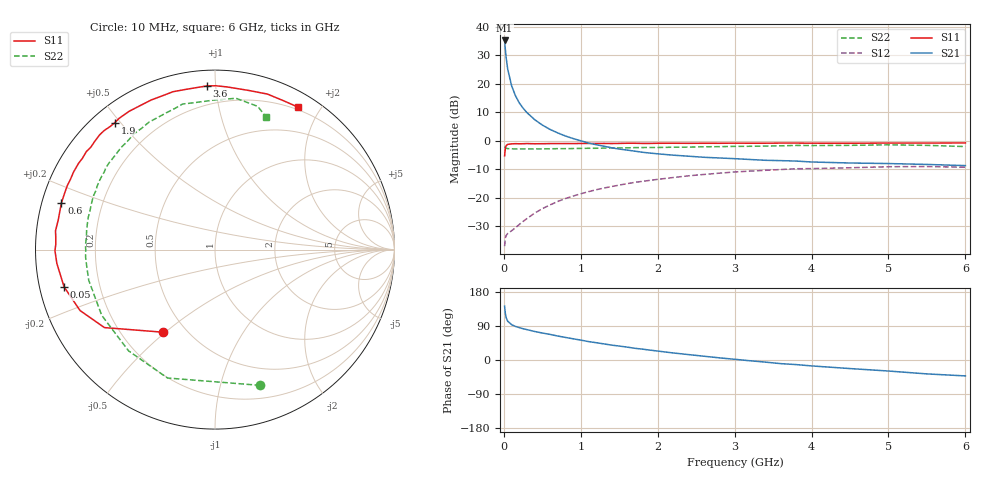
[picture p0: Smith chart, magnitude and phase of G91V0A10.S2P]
! SIEMENS Small Signal Semiconductors
! BFG235
! Si NPN RF Bipolar Junction Transistor in SOT223
! VCE = 1 V  IC = 100 mA
! Common Emitter S-Parameters:  July  1994
# GHz  S  MA  R  50
!  f  S11  S21  S12  S22
! GHz  MAG  ANG  MAG  ANG  MAG  ANG  MAG  ANG
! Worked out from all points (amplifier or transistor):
!   40 points, 10 MHz to 6 GHz, reference 50 ohm
!   highest |S21| = 35.1 dB at 10 MHz (marker M1)
!   |S21| within 3 dB of that: start of sweep to 19.22 MHz
!   unconditionally stable (mu >= 1): 411.8 MHz to 1.695 GHz; 1.703 GHz to 1.978 GHz
!   at 200 MHz: K = 0.80, MSG = 21.3 dB, |S12| = -29.3 dB
!   at 1.5 GHz: K = 1.02, MAG = 5.3 dB, |S12| = -15.5 dB
!   at 6 GHz: K = 0.95, MSG = 0.3 dB, |S12| = -9.3 dB
!   S11 on the Smith chart (normalised r, x): 10 MHz: 0.37, -0.49; 50 MHz: 0.07, -0.12; 600 MHz: 0.06, +0.15; 1.9 GHz: 0.06, +0.48; 3.6 GHz: 0.09, +0.95; 6 GHz: 0.17, +1.72
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0.01  0.5449 -122.4  57.2 141.9  0.0143 52.4  0.7971 -71.6
0.02  0.7538 -144.8  39.32 122.0  0.0199 37.1  0.7628 -110.3
0.03  0.825 -155.7  28.62 111.8  0.022 31.0  0.7417 -130.5
0.05  0.866 -166.1  18.09 102.3  0.0238 26.5  0.7297 -149.9
0.1  0.8845 -175.0  9.295 93.4  0.0266 31.4  0.724 -166.3
0.15  0.8917 -179.6  6.203 88.7  0.0299 38.8  0.7208 -173.0
0.2  0.8875 178.1  4.636 85.5  0.0342 43.9  0.7222 -176.8
0.25  0.8901 175.4  3.734 82.5  0.0388 48.7  0.7202 -179.6
0.3  0.8948 173.3  3.121 80.2  0.0435 51.3  0.7218 177.9
0.4  0.8888 169.3  2.353 75.3  0.0541 55.1  0.7202 174.3
0.5  0.8907 165.8  1.889 71.2  0.0648 56.7  0.7234 171.3
0.6  0.8943 163.1  1.585 67.6  0.0754 57.1  0.7257 168.3
0.8  0.8969 156.6  1.216 59.6  0.0974 56.2  0.7289 163.0
1.1  0.8994 147.7  0.916 48.6  0.1287 52.3  0.7404 155.9
1.4  0.8969 140.5  0.756 39.3  0.1581 47.3  0.7492 149.3
1.9  0.9011 128.3  0.61 26.1  0.2033 38.1  0.7633 138.6
2.2  0.907 121.8  0.561 18.6  0.2276 32.3  0.7728 132.7
3.2  0.9074 100.7  0.471 -2.0  0.2949 13.0  0.8018 113.9
3.6  0.9129 92.9  0.45 -9.6  0.3143 4.7  0.8179 105.8
4.5  0.9064 78.0  0.409 -22.6  0.3377 -10.7  0.833 90.5
5.5  0.9131 65.2  0.386 -36.7  0.3548 -28.0  0.8328 73.4
6  0.9185 59.9  0.368 -42.0  0.3447 -34.4  0.7932 69.1
